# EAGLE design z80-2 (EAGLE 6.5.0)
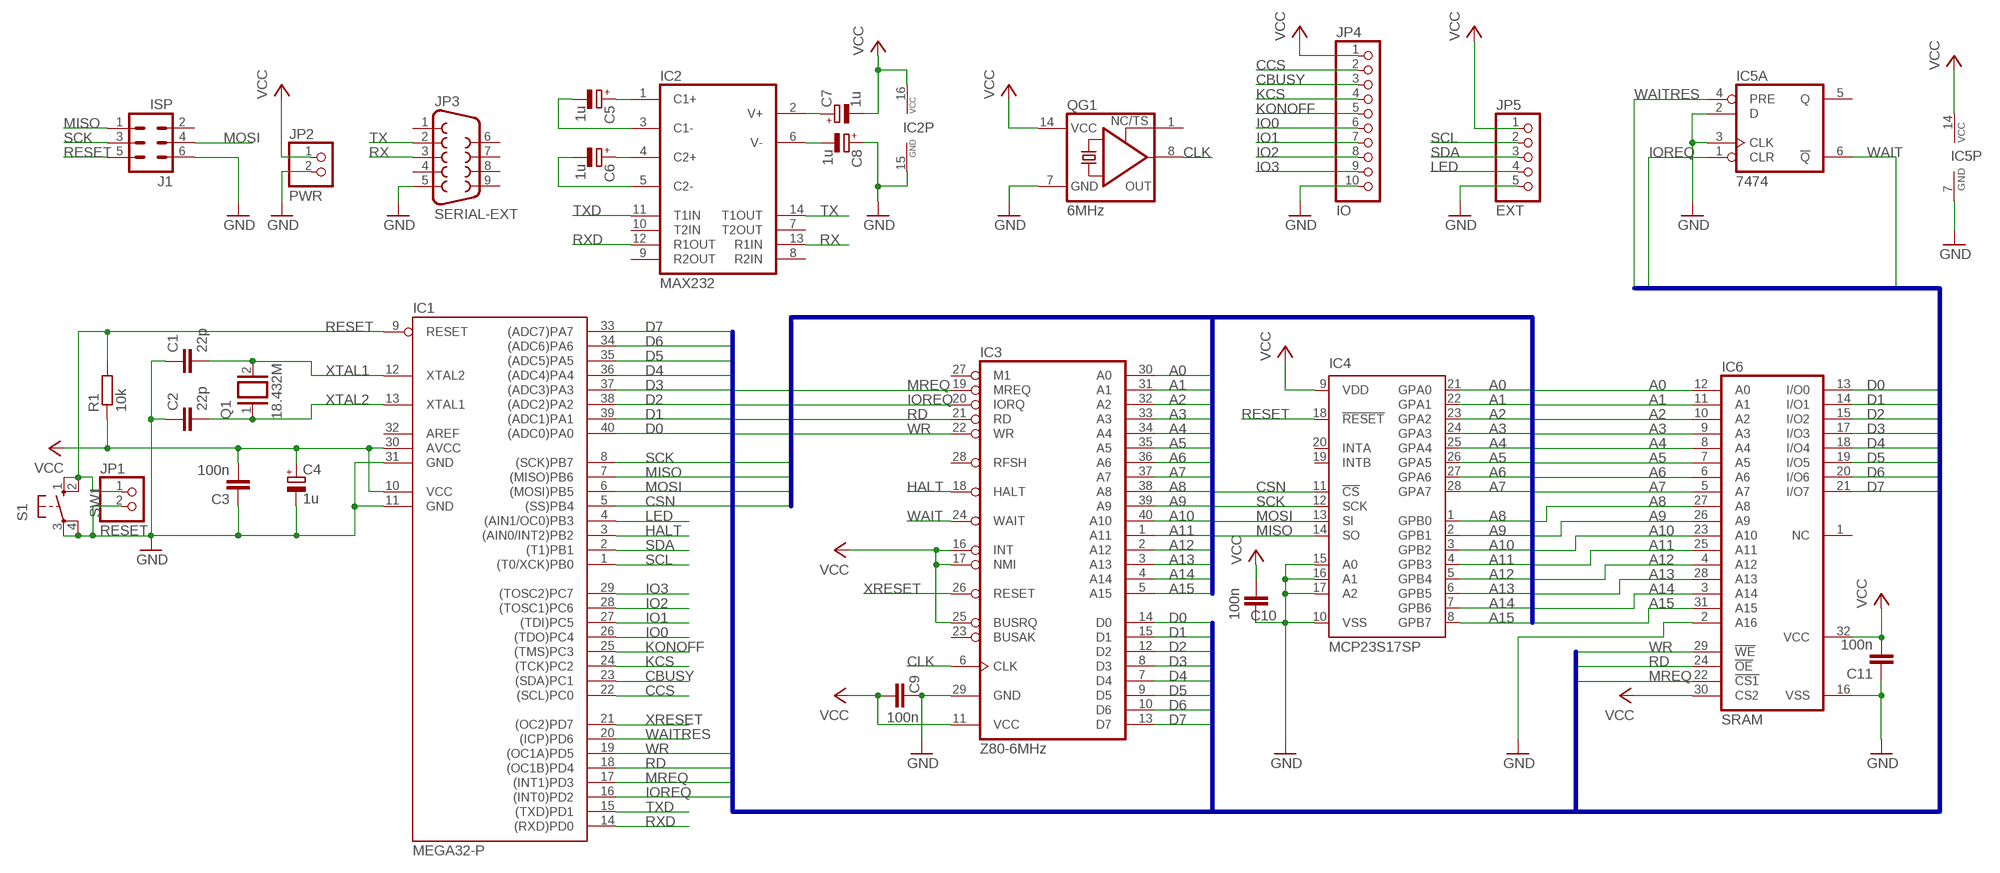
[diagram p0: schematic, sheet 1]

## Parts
C1  22p  C-EU025-024X044  [C025-024X044]
C2  22p  C-EU025-024X044  [C025-024X044]
C3  100n  C-EU025-024X044  [C025-024X044]
C4  1u  CPOL-EUE2.5-5  [E2,5-5]
C5  1u  CPOL-EUE2-5  [E2-5]
C6  1u  CPOL-EUE2.5-5  [E2,5-5]
C7  1u  CPOL-EUE2.5-5  [E2,5-5]
C8  1u  CPOL-EUE2.5-5  [E2,5-5]
C9  100n  C-EU025-024X044  [C025-024X044]
C10  100n  C-EU025-024X044  [C025-024X044]
C11  100n  C-EU025-024X044  [C025-024X044]
IC1  MEGA32-P  [DIL40]
IC2  MAX232  [DIL16]
IC3  Z80-6MHz  Z80CPU  [DIL40]
IC4  MCP23S17SP  [DIL28-3]
IC5  7474  74S74N  [DIL14]
IC6  SRAM  628128P  [DIL32]
J1  ISP  ML6L  [ML6L]
JP1  RESET  PINHD-1X2  [1X02]
JP2  PWR  PINHD-1X2  [1X02]
JP3  SERIAL-EXT  F09HP  [F09HP]
JP4  IO  PINHD-1X10  [1X10]
JP5  EXT  PINHD-1X5  [1X05]
Q1  18.432M  XTAL/S  [QS]
QG1  6MHz  XO-14  [DIL14S]
R1  10k  R-EU_0207/10  [0207/10]
S1  SW1  10-XX  [B3F-10XX]

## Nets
A0: IC3.30(A0) IC4.21(GPA0) IC6.12(A0)
A1: IC3.31(A1) IC4.22(GPA1) IC6.11(A1)
A2: IC3.32(A2) IC4.23(GPA2) IC6.10(A2)
A3: IC3.33(A3) IC4.24(GPA3) IC6.9(A3)
A4: IC3.34(A4) IC4.25(GPA4) IC6.8(A4)
A5: IC3.35(A5) IC4.26(GPA5) IC6.7(A5)
A6: IC3.36(A6) IC4.27(GPA6) IC6.6(A6)
A7: IC3.37(A7) IC4.28(GPA7) IC6.5(A7)
A8: IC3.38(A8) IC4.1(GPB0) IC6.27(A8)
A9: IC3.39(A9) IC4.2(GPB1) IC6.26(A9)
A10: IC3.40(A10) IC4.3(GPB2) IC6.23(A10)
A11: IC3.1(A11) IC4.4(GPB3) IC6.25(A11)
A12: IC3.2(A12) IC4.5(GPB4) IC6.4(A12)
A13: IC3.3(A13) IC4.6(GPB5) IC6.28(A13)
A14: IC3.4(A14) IC4.7(GPB6) IC6.3(A14)
A15: IC3.5(A15) IC4.8(GPB7) IC6.31(A15)
CBUSY: IC1.23((SDA)PC1) JP4.3
CCS: IC1.22((SCL)PC0) JP4.2
CLK: IC3.6(CLK) QG1.8(OUT)
CSN: IC1.5((SS)PB4) IC4.11(!CS)
D0: IC1.40((ADC0)PA0) IC3.14(D0) IC6.13(I/O0)
D1: IC1.39((ADC1)PA1) IC3.15(D1) IC6.14(I/O1)
D2: IC1.38((ADC2)PA2) IC3.12(D2) IC6.15(I/O2)
D3: IC1.37((ADC3)PA3) IC3.8(D3) IC6.17(I/O3)
D4: IC1.36((ADC4)PA4) IC3.7(D4) IC6.18(I/O4)
D5: IC1.35((ADC5)PA5) IC3.9(D5) IC6.19(I/O5)
D6: IC1.34((ADC6)PA6) IC3.10(D6) IC6.20(I/O6)
D7: IC1.33((ADC7)PA7) IC3.13(D7) IC6.21(I/O7)
GND: C1.1 C2.1 C3.1 C4.- C8.+ C9.1 C10.1 C11.1 IC1.11(GND) IC1.31(GND) IC2.15(GND) IC3.29(GND) IC4.10(VSS) IC4.15(A0) IC4.16(A1) IC4.17(A2) IC5.2(A:D) IC5.3(A:CLK) IC5.7(P:GND) IC6.2(A16) IC6.16(VSS) J1.6 JP1.2 JP2.2 JP3.5 JP4.10 JP5.5 QG1.7(GND) S1.3(P) S1.4(P1)
HALT: IC1.3((AIN0/INT2)PB2) IC3.18(HALT)
IO0: IC1.26((TDO)PC4) JP4.6
IO1: IC1.27((TDI)PC5) JP4.7
IO2: IC1.28((TOSC1)PC6) JP4.8
IO3: IC1.29((TOSC2)PC7) JP4.9
IOREQ: IC1.16((INT0)PD2) IC3.20(IORQ) IC5.1(A:CLR)
KCS: IC1.24((TCK)PC2) JP4.4
KONOFF: IC1.25((TMS)PC3) JP4.5
LED: IC1.4((AIN1/OC0)PB3) JP5.4
MISO: IC1.7((MISO)PB6) IC4.14(SO) J1.1
MOSI: IC1.6((MOSI)PB5) IC4.13(SI) J1.4
MREQ: IC1.17((INT1)PD3) IC3.19(MREQ) IC6.22(!CS1)
N$21: C5.+ IC2.1(C1+)
N$22: C6.+ IC2.4(C2+)
N$23: C5.- IC2.3(C1-)
N$24: C6.- IC2.5(C2-)
N$28: C7.+ IC2.2(V+)
N$29: C8.- IC2.6(V-)
RD: IC1.18((OC1B)PD4) IC3.21(RD) IC6.24(!OE)
RESET: IC1.9(RESET) IC4.18(!RESET) J1.5 JP1.1 R1.2 S1.1(S) S1.2(S1)
RX: IC2.13(R1IN) JP3.3
RXD: IC1.14((RXD)PD0) IC2.12(R1OUT)
SCK: IC1.8((SCK)PB7) IC4.12(SCK) J1.3
SCL: IC1.1((T0/XCK)PB0) JP5.2
SDA: IC1.2((T1)PB1) JP5.3
TX: IC2.14(T1OUT) JP3.2
TXD: IC1.15((TXD)PD1) IC2.11(T1IN)
VCC: C3.2 C4.+ C7.- C9.2 C10.2 C11.2 IC1.10(VCC) IC1.30(AVCC) IC2.16(VCC) IC3.11(VCC) IC3.16(INT) IC3.17(NMI) IC3.25(BUSRQ) IC4.9(VDD) IC5.14(P:VCC) IC6.30(CS2) IC6.32(VCC) JP2.1 JP4.1 JP5.1 QG1.14(VCC) R1.1
WAIT: IC3.24(WAIT) IC5.6(A:!Q)
WAITRES: IC1.20((ICP)PD6) IC5.4(A:PRE)
WR: IC1.19((OC1A)PD5) IC3.22(WR) IC6.29(!WE)
XRESET: IC1.21((OC2)PD7) IC3.26(RESET)
XTAL1: C1.2 IC1.12(XTAL2) Q1.2
XTAL2: C2.2 IC1.13(XTAL1) Q1.1
Unconnected: IC1.32(AREF) IC2.7(T2OUT) IC2.8(R2IN) IC2.9(R2OUT) IC2.10(T2IN) IC3.23(BUSAK) IC3.27(M1) IC3.28(RFSH) IC4.19(INTB) IC4.20(INTA) IC5.5(A:Q) IC5.8(B:!Q) IC5.9(B:Q) IC5.10(B:PRE) IC5.11(B:CLK) IC5.12(B:D) IC5.13(B:CLR) IC6.1(NC) J1.2 JP3.1 JP3.4 JP3.6 JP3.7 JP3.8 JP3.9 QG1.1(TS)

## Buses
BUS_ADDR:A[0..15],SCK,MISO,MOSI,CSN
BUD_DAT:D[0..7],RD,WR,MREQ,IOREQ,WAITRES,WAIT

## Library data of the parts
C1-C3 C9-C11 = rcl:C-EU: CAPACITOR, European symbol
C4-C8 = rcl:CPOL-EU: POLARIZED CAPACITOR, European symbol
IC1 = atmel:MEGA32-P: MICROCONTROLLER 32 Kbytes FLASH 2 Kbytes SRAM 1 Kbytes EEPROM USART 8-channel 10 bit ADC Source: www.atmel.com .. doc2503.pdf; MPN: ATMEGA32-16PU; OC_FARNELL: 1661729; OC_NEWARK: 51P1794
IC2 = maxim:MAX232: RS232 TRANSCEIVER; MF: MAXIM; MPN: MAX232ACPE+; OC_FARNELL: 9723773; OC_NEWARK: 68K4544
IC3 = zilog:Z80CPU: Z80 FAMILY DEVICE
IC4 = microchip:MCP23S17: http://ww1.microchip.com/downloads/en/DeviceDoc/21952a.pdf Source: http://ww1.microchip.com/downloads/en/DeviceDoc/21952a.pdf; MF: MICROCHIP; MPN: MCP23S17-E/SP; OC_FARNELL: 1292238; OC_NEWARK: 31K2951
IC5 = 74xx-eu:74*74: Dual D type positive edge triggered FLIP FLOP, preset and clear
IC6 = memory-hitachi:628128P: MEMORY
J1 = con-harting-ml:ML6: HARTING; OC_FARNELL: unknown; OC_NEWARK: unknown
JP1 JP2 = pinhead:PINHD-1X2: PIN HEADER
JP3 = con-subd:F09: SUB-D; OC_FARNELL: unknown; OC_NEWARK: unknown
JP4 = pinhead:PINHD-1X10: PIN HEADER
JP5 = pinhead:PINHD-1X5: PIN HEADER
Q1 = special:XTAL/S: CRYSTAL
QG1 = crystal:XO-: CRYSTAL; OC_FARNELL: unknown; OC_NEWARK: unknown
R1 = rcl:R-EU_: RESISTOR, European symbol
S1 = switch-omron:10-XX: OMRON SWITCH; MPN: B3F-1000; OC_FARNELL: 176432; OC_NEWARK: 36M3542

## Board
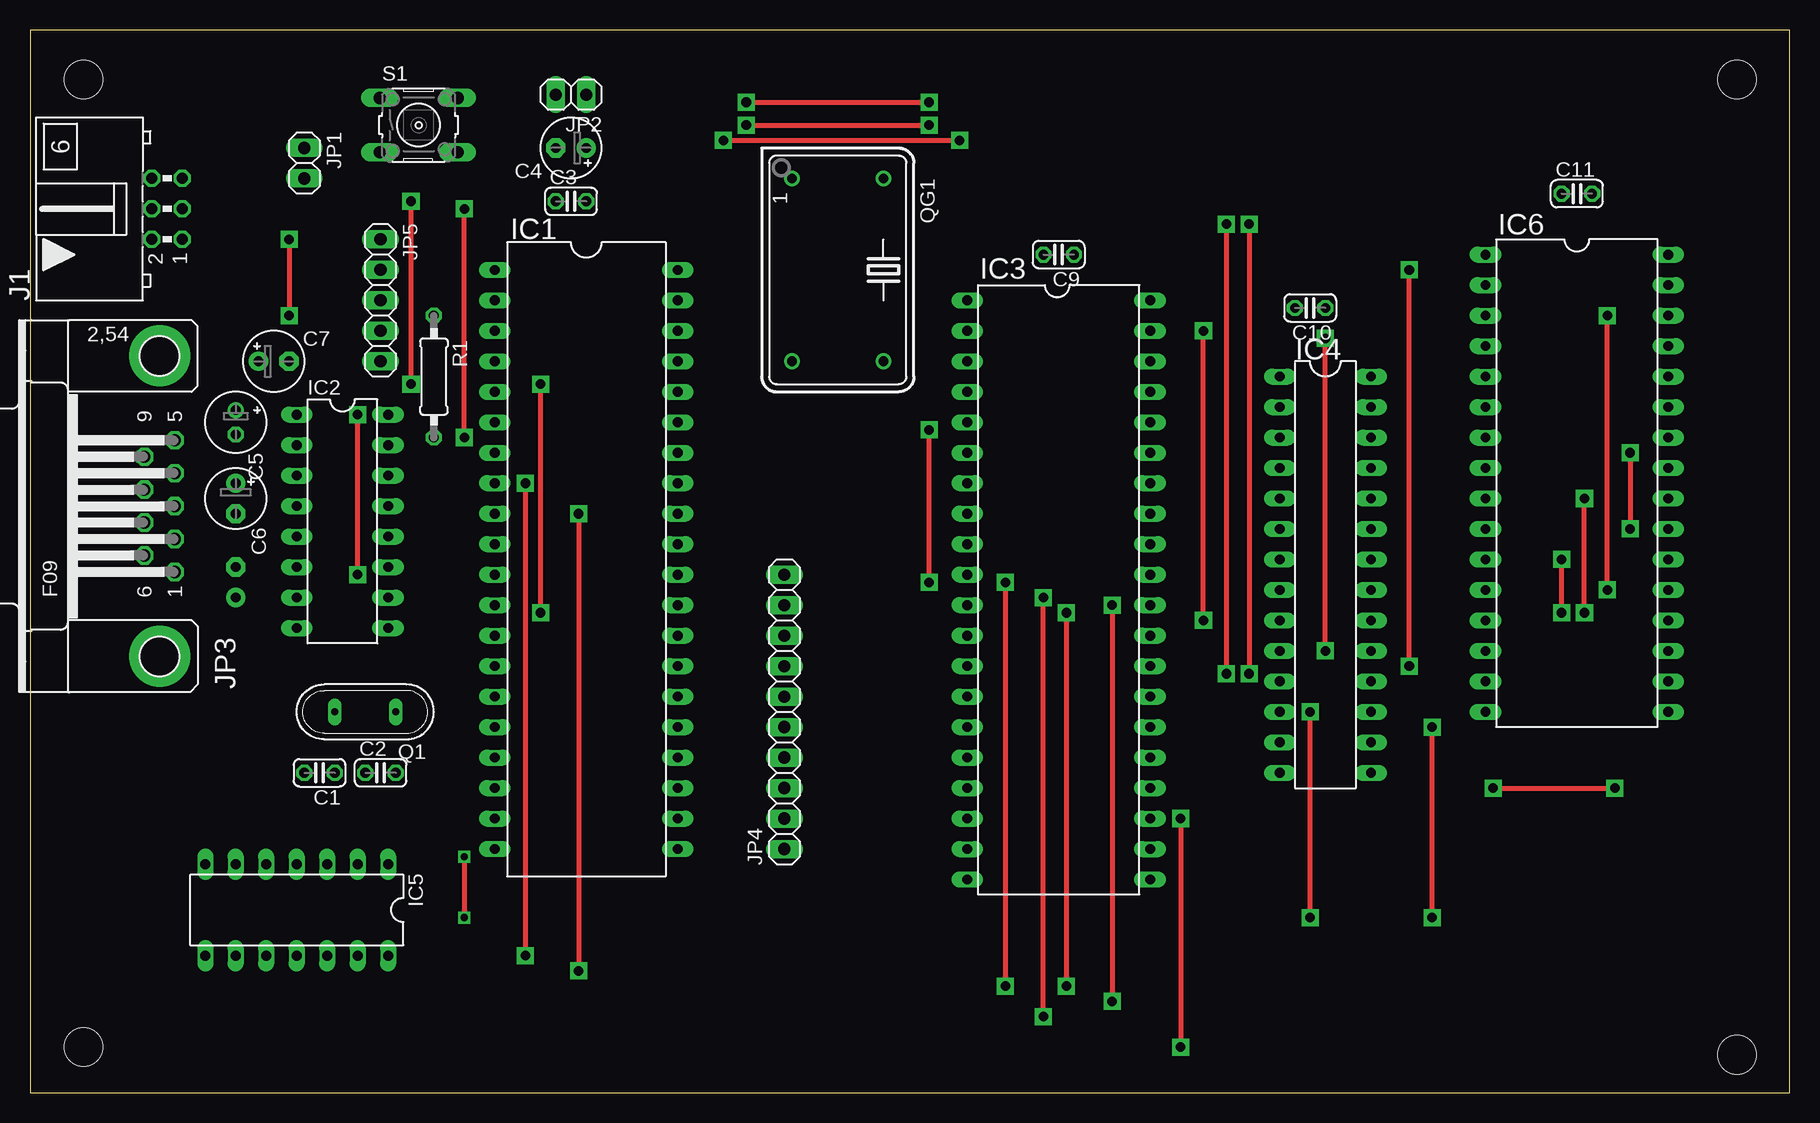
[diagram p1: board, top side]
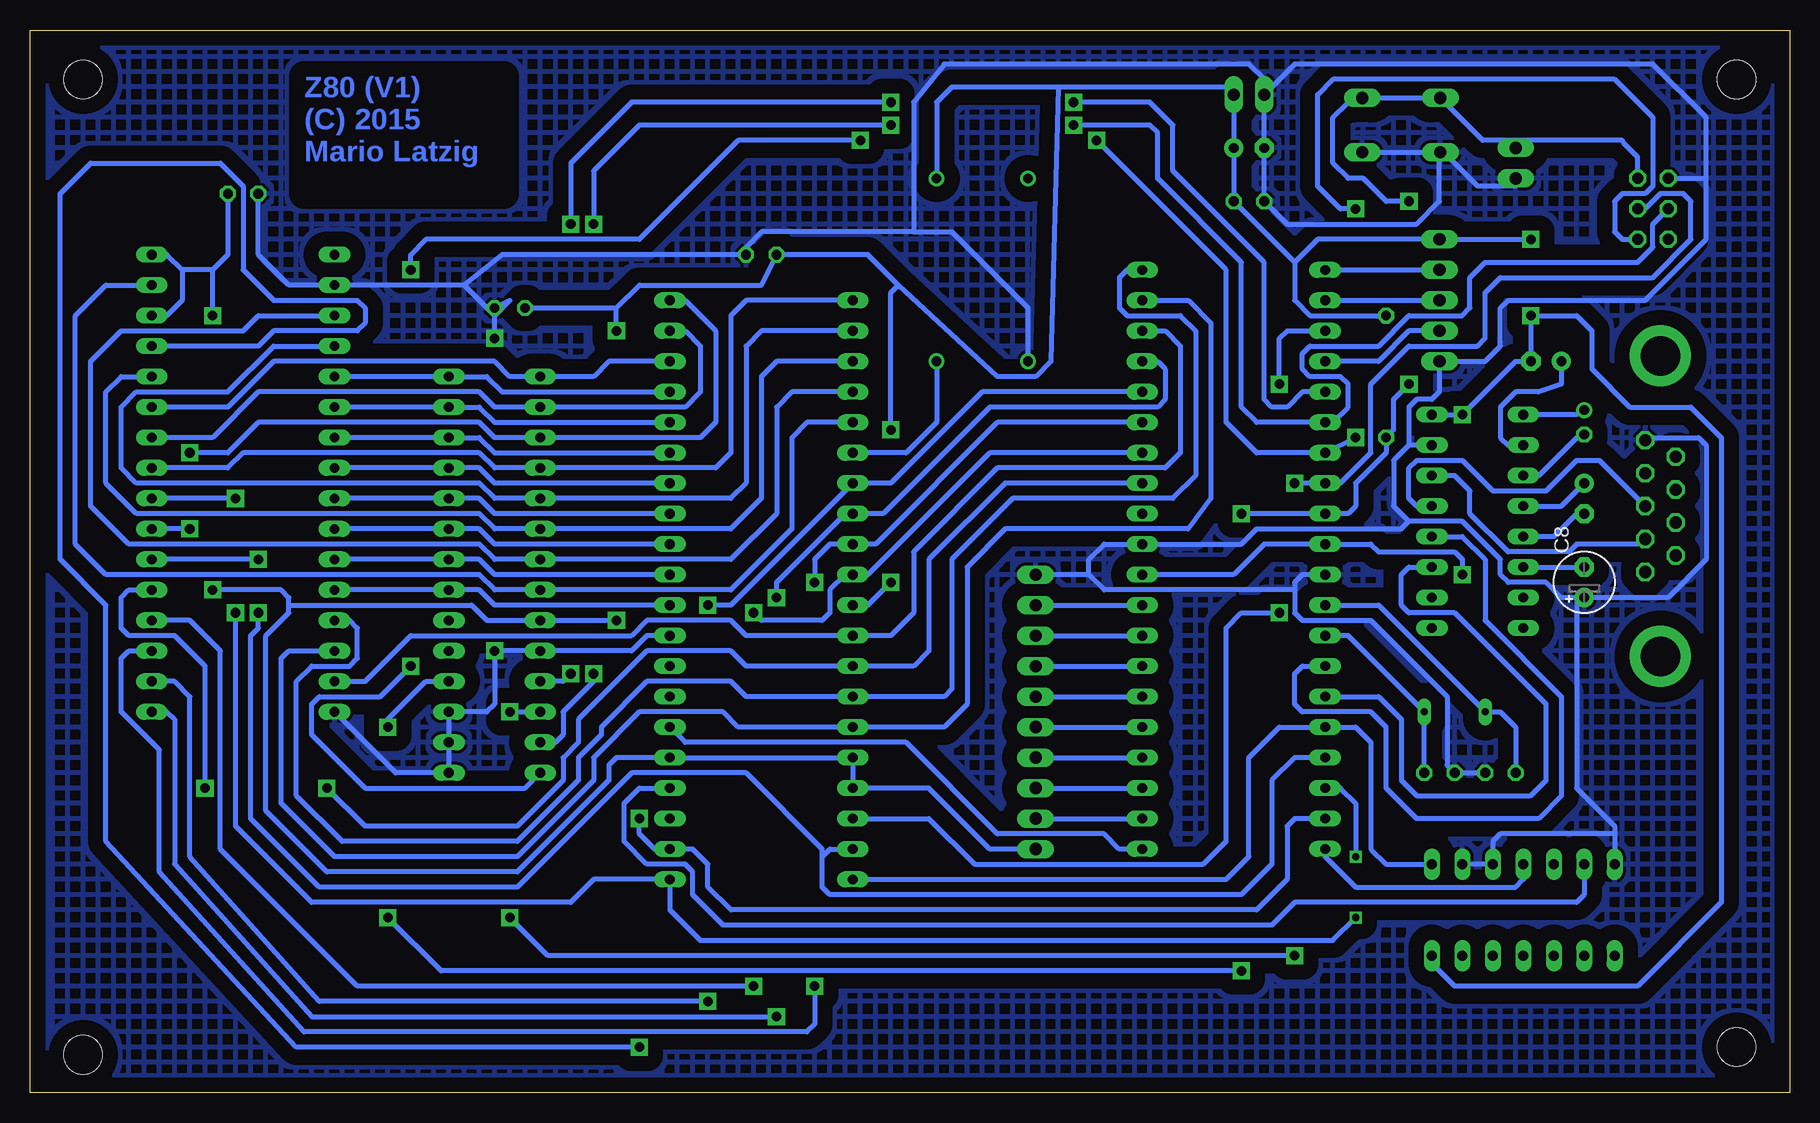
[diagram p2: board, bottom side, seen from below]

Size 146.66 x 88.57 mm. Coordinates in mm from the lower left corner, seen from the top.
Outline: 0,0 146.66,0 146.66,88.57 0,88.57 0,0
Copper layers (1*16): Top 0.035mm / dielectric 1.5mm / Bottom 0.035mm
Design rules "platinenbelichter": minimum track width 10mil, minimum drill 24mil, track to track 10mil, track to pad 10mil, pad to pad 10mil, via to via 10mil, smd to smd 10mil, copper to edge 40mil, drill to drill 8mil, minimum pad ring 10mil, minimum via ring 8mil, stop-mask expansion 10mil, vias tented up to drill 0mil, thermal gap 10mil
Holes 3.2 mm at 4.45,84.45 4.45,3.81 142.24,3.17 142.24,84.45

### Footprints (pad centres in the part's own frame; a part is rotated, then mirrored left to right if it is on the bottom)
C025-024X044 = drill 0.813 octagon: 1 -1.27,0; 2 1.27,0
E2,5-5 = drill 0.813 pad 1.6: + -1.27,0 | drill 0.813 pad 1.6 octagon: - 1.27,0
E2-5 = drill 0.813 pad 1.27: + -1.016,0 | drill 0.813 pad 1.27 octagon: - 1.016,0
DIL40 = drill 0.813 long: 1 -24.13,-7.62; 2 -21.59,-7.62; 3 -19.05,-7.62; 4 -16.51,-7.62; 5 -13.97,-7.62; 6 -11.43,-7.62; 7 -8.89,-7.62; 8 -6.35,-7.62; 9 -3.81,-7.62; 10 -1.27,-7.62; 11 1.27,-7.62; 12 3.81,-7.62; 13 6.35,-7.62; 14 8.89,-7.62; 15 11.43,-7.62; 16 13.97,-7.62; 17 16.51,-7.62; 18 19.05,-7.62; 19 21.59,-7.62; 20 24.13,-7.62; 21 24.13,7.62; 22 21.59,7.62; 23 19.05,7.62; 24 16.51,7.62; 25 13.97,7.62; 26 11.43,7.62; 27 8.89,7.62; 28 6.35,7.62; 29 3.81,7.62; 30 1.27,7.62; 31 -1.27,7.62; 32 -3.81,7.62; 33 -6.35,7.62; 34 -8.89,7.62; 35 -11.43,7.62; 36 -13.97,7.62; 37 -16.51,7.62; 38 -19.05,7.62; 39 -21.59,7.62; 40 -24.13,7.62
DIL16 = drill 0.813 long: 1 -8.89,-3.81; 2 -6.35,-3.81; 3 -3.81,-3.81; 4 -1.27,-3.81; 5 1.27,-3.81; 6 3.81,-3.81; 7 6.35,-3.81; 8 8.89,-3.81; 9 8.89,3.81; 10 6.35,3.81; 11 3.81,3.81; 12 1.27,3.81; 13 -1.27,3.81; 14 -3.81,3.81; 15 -6.35,3.81; 16 -8.89,3.81
DIL28-3 = drill 0.813 long: 1 -16.51,-3.81; 2 -13.97,-3.81; 3 -11.43,-3.81; 4 -8.89,-3.81; 5 -6.35,-3.81; 6 -3.81,-3.81; 7 -1.27,-3.81; 8 1.27,-3.81; 9 3.81,-3.81; 10 6.35,-3.81; 11 8.89,-3.81; 12 11.43,-3.81; 13 13.97,-3.81; 14 16.51,-3.81; 15 16.51,3.81; 16 13.97,3.81; 17 11.43,3.81; 18 8.89,3.81; 19 6.35,3.81; 20 3.81,3.81; 21 1.27,3.81; 22 -1.27,3.81; 23 -3.81,3.81; 24 -6.35,3.81; 25 -8.89,3.81; 26 -11.43,3.81; 27 -13.97,3.81; 28 -16.51,3.81
DIL14 = drill 0.813 long: 1 -7.62,-3.81; 2 -5.08,-3.81; 3 -2.54,-3.81; 4 0,-3.81; 5 2.54,-3.81; 6 5.08,-3.81; 7 7.62,-3.81; 8 7.62,3.81; 9 5.08,3.81; 10 2.54,3.81; 11 0,3.81; 12 -2.54,3.81; 13 -5.08,3.81; 14 -7.62,3.81
DIL32 = drill 0.813 long: 1 -19.05,-7.62; 2 -16.51,-7.62; 3 -13.97,-7.62; 4 -11.43,-7.62; 5 -8.89,-7.62; 6 -6.35,-7.62; 7 -3.81,-7.62; 8 -1.27,-7.62; 9 1.27,-7.62; 10 3.81,-7.62; 11 6.35,-7.62; 12 8.89,-7.62; 13 11.43,-7.62; 14 13.97,-7.62; 15 16.51,-7.62; 16 19.05,-7.62; 17 19.05,7.62; 18 16.51,7.62; 19 13.97,7.62; 20 11.43,7.62; 21 8.89,7.62; 22 6.35,7.62; 23 3.81,7.62; 24 1.27,7.62; 25 -1.27,7.62; 26 -3.81,7.62; 27 -6.35,7.62; 28 -8.89,7.62; 29 -11.43,7.62; 30 -13.97,7.62; 31 -16.51,7.62; 32 -19.05,7.62
ML6L = drill 0.914 octagon: 1 -2.54,-1.27; 2 -2.54,1.27; 3 0,-1.27; 4 0,1.27; 5 2.54,-1.27; 6 2.54,1.27
1X02 = drill 1.016 long: 1 -1.27,0; 2 1.27,0
F09HP = drill 1.016 octagon: 1 -5.486,-1.27; 2 -2.743,-1.27; 3 0,-1.27; 4 2.743,-1.27; 5 5.486,-1.27; 6 -4.115,1.27; 7 -1.372,1.27; 8 1.372,1.27; 9 4.115,1.27 | drill 3.302 pad 5.08: G1 -12.522,0; G2 12.522,0
1X10 = drill 1.016 long: 1 -11.43,0; 2 -8.89,0; 3 -6.35,0; 4 -3.81,0; 5 -1.27,0; 6 1.27,0; 7 3.81,0; 8 6.35,0; 9 8.89,0; 10 11.43,0
1X05 = drill 1.016 long: 1 -5.08,0; 2 -2.54,0; 3 0,0; 4 2.54,0; 5 5.08,0
QS = drill 0.61 long: 1 -2.54,0; 2 2.54,0
DIL14S = drill 0.813: 1 -7.62,-3.81; 7 7.62,-3.81; 8 7.62,3.81; 14 -7.62,3.81
0207/10 = drill 0.813 octagon: 1 -5.08,0; 2 5.08,0
B3F-10XX = drill 1.016 long: 1 -3.251,2.261; 2 3.251,2.261; 3 -3.251,-2.261; 4 3.251,-2.261

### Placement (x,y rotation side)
C1  24.13,26.67 180 top
C2  29.21,26.67 0 top
C3  45.09,74.3 0 top
C4  45.09,78.74 180 top
C5  17.14,55.88 270 top
C6  17.14,49.53 270 top
C7  20.32,60.96 0 top
C8  17.14,42.55 90 bottom
C9  85.72,69.85 180 top
C10  106.68,65.41 180 top
C11  128.91,74.93 0 top
IC1  46.35,44.45 270 top
IC2  26.04,47.62 270 top
IC3  85.72,41.91 270 top
IC4  107.95,43.18 270 top
IC5  22.23,15.24 180 top
IC6  128.91,50.8 270 top
J1  11.43,73.66 90 top
JP1  22.86,77.47 270 top
JP2  45.09,83.19 180 top
JP3  10.79,48.9 90 top
JP4  62.87,31.75 90 top
JP5  29.21,66.04 270 top
Q1  27.94,31.75 180 top
QG1  67.31,68.58 270 top
R1  33.66,59.69 270 top
S1  32.38,80.64 0 top

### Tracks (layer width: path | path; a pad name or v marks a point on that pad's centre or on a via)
A0
  Bottom 0.406: IC6.12 IC4.21 109.22,41.91 107.95,40.64 IC3.30
A1
  Bottom 0.406: IC6.11 IC4.22 109.22,44.45 107.95,43.18 IC3.31
A2
  Bottom 0.406: IC6.10 IC4.23 109.22,46.99 107.95,45.72 IC3.32
A3
  Bottom 0.406: IC6.9 IC4.24 109.22,49.53 107.95,48.26 IC3.33
A4
  Bottom 0.406: IC6.8 IC4.25 109.22,52.07 107.95,50.8 IC3.34
A5
  Bottom 0.406: IC6.7 IC4.26 109.22,54.61 107.95,53.34 IC3.35
A6
  Bottom 0.406: IC6.6 IC4.27 109.22,57.15 107.95,55.88 IC3.36
A7
  Bottom 0.406: IC6.5 IC4.28 108.58,59.69 107.31,58.42 IC3.37
A8
  Bottom 0.406: IC3.38 98.42,60.96 99.69,59.69 IC4.1 106.68,59.69 107.95,60.96 126.36,60.96 130.18,57.15 IC6.27
A9
  Bottom 0.406: IC3.39 92.08,63.5 90.81,62.23 90.81,58.42 92.08,57.15 IC4.2 107.95,57.15 109.22,58.42 127.64,58.42 131.44,54.61 IC6.26
A10  (via drill 0.8 pad 1.42)
  Top 0.406: v133.35,53.34 v133.35,46.99
  Bottom 0.406: IC3.40 92.08,66.04 89.53,63.5 89.53,55.88 90.81,54.61 IC4.3 107.95,54.61 109.22,55.88 127.64,55.88 130.18,53.34 v133.35,53.34 | v133.35,46.99 IC6.23
A11
  Bottom 0.406: IC3.1 87,66.04 88.27,64.77 88.27,53.34 89.53,52.07 IC4.4 107.95,52.07 109.22,53.34 128.91,53.34 130.18,52.07 IC6.25
A12
  Bottom 0.406: IC3.2 85.72,63.5 87,62.23 87,50.8 88.27,49.53 IC4.5 107.95,49.53 109.22,50.8 137.79,50.8 139.06,52.07 139.06,57.15 137.79,58.42 130.18,58.42 126.36,62.23 IC6.4
A13
  Bottom 0.406: IC3.3 84.45,60.96 85.72,59.69 85.72,49.53 88.27,46.99 IC4.6 107.95,46.99 109.22,48.26 137.79,48.26 140.34,50.8 140.34,58.42 139.06,59.69 IC6.28
A14
  Bottom 0.406: IC3.4 83.19,58.42 84.45,57.15 84.45,48.26 88.27,44.45 IC4.7 107.95,44.45 109.22,45.72 138.43,45.72 141.6,48.9 141.6,60.96 139.06,63.5 128.91,63.5 127.64,64.77 IC6.3
A15
  Bottom 0.406: IC3.5 81.92,55.88 83.19,54.61 83.19,46.99 88.27,41.91 IC4.8 107.95,41.91 109.22,43.18 140.34,43.18 142.88,45.72 142.88,64.77 140.34,67.31 IC6.31
CBUSY
  Bottom 0.406: JP4.3 IC1.23
CCS
  Bottom 0.406: JP4.2 IC1.22
CLK
  Bottom 0.406: QG1.8 71.12,55.88 73.66,53.34 IC3.6
CSN  (via drill 0.8 pad 1.42)
  Top 0.406: v59.69,82.55 v74.93,82.55 | v101.6,72.39 v101.6,34.92
  Bottom 0.406: IC1.5 40.64,58.42 41.91,57.15 43.18,57.15 43.81,57.78 43.81,69.22 51.44,76.83 51.44,80.64 53.34,82.55 v59.69,82.55 | v74.93,82.55 96.52,82.55 101.6,77.47 v101.6,72.39 | v101.6,34.92 102.23,34.29 IC4.11
D0
  Bottom 0.406: IC6.13 120.02,39.37 119.38,38.73 119.38,36.2 120.02,35.56 123.19,35.56 124.46,34.29 124.46,24.77 120.65,20.95 106.05,20.95 100.97,26.04 100.97,27.94 99.06,29.84 99.06,30.48 95.25,34.29 88.27,34.29 87,33.02 IC3.14 70.48,33.02 69.85,33.66 69.85,44.45 64.77,49.53 51.44,49.53 49.53,51.44 49.53,63.5 50.8,64.77 55.24,64.77 55.88,65.41 55.88,67.94 55.24,68.58 IC1.40
D1
  Bottom 0.406: IC6.14 125.09,36.83 125.73,36.2 125.73,24.13 121.28,19.68 106.05,19.68 99.69,26.04 99.69,27.94 95.89,31.75 88.9,31.75 87.63,30.48 IC3.15 70.48,30.48 68.58,32.38 68.58,43.81 65.41,46.99 50.16,46.99 48.26,49.53 48.26,64.14 50.16,66.04 IC1.39
D2
  Bottom 0.406: IC1.38 52.07,63.5 50.8,62.23 50.8,53.34 52.07,52.07 66.04,52.07 73.03,45.09 73.03,40.01 74.93,38.1 IC3.12 87,38.1 88.27,39.37 95.25,39.37 96.52,38.1 114.94,38.1 118.75,34.29 IC6.15
D3  (via drill 0.8 pad 1.42)
  Top 0.406: v84.45,6.35 v84.45,41.27
  Bottom 0.406: IC6.17 135.25,31.75 134.62,31.11 134.62,19.05 123.19,6.35 v84.45,6.35 | v84.45,41.27 84.45,42.55 78.74,48.26 IC3.8 75.56,48.26 66.67,57.15 52.7,57.15 52.07,57.78 52.07,60.33 52.7,60.96 IC1.37
D4  (via drill 0.8 pad 1.42)
  Top 0.406: v90.17,40.64 v90.17,7.62
  Bottom 0.406: v90.17,40.64 88.27,40.64 IC3.7 74.93,50.8 67.31,58.42 IC1.36 | v90.17,7.62 122.56,7.62 133.35,19.68 133.35,33.02 134.62,34.29 IC6.18
D5  (via drill 0.8 pad 1.42)
  Top 0.406: v81.28,42.55 v81.28,8.89
  Bottom 0.406: v81.28,42.55 81.28,44.45 80.01,45.72 IC3.9 76.2,45.72 66.04,55.88 IC1.35 | v81.28,8.89 81.28,5.71 81.92,5.08 123.83,5.08 135.89,18.41 135.89,28.57 139.06,31.75 139.06,36.2 138.43,36.83 IC6.19
D6  (via drill 0.8 pad 1.42)
  Top 0.406: v86.36,40.01 v86.36,8.89
  Bottom 0.406: v86.36,40.01 85.72,39.37 80.64,39.37 80.01,40.01 80.01,41.91 78.74,43.18 IC3.10 76.83,43.18 66.67,53.34 IC1.34 | v86.36,8.89 119.38,8.89 130.81,20.32 130.81,36.83 133.35,39.37 IC6.20
D7  (via drill 0.8 pad 1.42)
  Top 0.406: v121.92,25.4 v132.08,25.4
  Bottom 0.406: v121.92,25.4 118.75,22.23 106.05,22.23 102.23,26.04 102.23,27.94 100.97,29.21 100.97,31.11 95.25,36.83 88.27,36.83 87,35.56 IC3.13 73.03,35.56 71.75,36.83 71.75,44.45 65.41,50.8 IC1.33 | v132.08,25.4 132.08,35.56 134.62,38.1 138.43,38.1 139.06,38.73 139.06,41.27 138.43,41.91 IC6.21
GND  (via drill 0.8 pad 1.42)
  Top 0.406: v107.95,36.83 v107.95,62.87
  Bottom 0.406: C11.1 127.64,69.85 125.09,67.31 IC6.2 110.49,67.31 | IC6.16 116.2,26.67 IC4.15 IC4.16 IC4.17 108.58,31.75 107.95,32.38 v107.95,36.83 IC4.10 96.52,36.83 95.25,38.1 IC3.29 | C1.1 C2.1 28.57,27.3 28.57,33.02 34.92,39.37 40.64,39.37 41.27,40.01 41.27,41.91 | IC1.11 40.64,43.18 41.27,42.55 41.27,41.91 | 17.78,41.27 C8.+ 10.16,41.27 6.99,44.45 6.99,53.98 7.62,54.61 11.43,54.61 JP3.5 | 17.78,41.27 19.05,41.27 20.32,42.55 23.5,42.55 24.13,43.18 24.13,44.45 27.3,47.62 31.75,47.62 | 31.75,47.62 32.38,46.99 44.45,46.99 45.72,45.72 IC1.31 57.15,45.72 58.42,44.45 58.42,43.18 | IC2.15 31.75,53.98 | 31.75,53.98 33.02,52.7 33.02,48.9 31.75,47.62 | 31.75,53.98 31.75,57.15 31.11,57.78 29.84,57.78 29.21,58.42 JP5.5 25.4,60.96 24.13,62.23 24.13,65.41 23.5,66.04 12.06,66.04 6.99,71.12 6.99,76.2 | S1.3 28.85,78.11 28.57,78.11 26.04,75.56 22.86,75.56 JP1.2 | JP2.2 C4.- C3.1 41.91,72.39 31.11,72.39 29.21,74.3 29.21,78.31 S1.3 | JP2.2 43.81,84.45 45.09,85.72 70.48,85.72 73.03,82.55 73.03,71.75 | 73.03,71.75 69.85,71.75 63.5,65.41 QG1.7 | S1.4 S1.3 | 6.99,76.2 6.99,81.28 11.43,85.72 41.27,85.72 JP2.2 | 41.27,41.91 57.15,41.91 58.42,43.18 | 58.42,43.18 JP4.10 | 73.03,71.75 85.72,71.75 87,70.48 C9.1 107.31,69.85 110.49,67.31 | v107.95,62.87 107.95,64.77 | 107.95,64.77 110.49,67.31 | C10.1 106.68,66.04 107.95,64.77 | J1.6 6.99,76.2 | 17.78,41.27 17.78,25.4 14.61,22.23 14.61,21.59 | 14.61,21.59 IC5.7 | 14.61,21.59 24.13,21.59 24.77,20.95 IC5.3 IC5.2
  pour Bottom (isolate 1.27, hatched): 146.69,88.9 146.69,0 0,0 0,88.9
HALT  (via drill 0.8 pad 1.42)
  Top 0.406: v42.55,40.01 v42.55,59.05
  Bottom 0.406: IC3.18 71.75,22.86 67.94,19.05 48.9,19.05 46.99,20.95 46.99,38.73 45.72,40.01 v42.55,40.01 | v42.55,59.05 42.55,62.87 41.91,63.5 IC1.3
IO0
  Bottom 0.406: JP4.6 IC1.26
IO1
  Bottom 0.406: JP4.7 IC1.27
IO2
  Bottom 0.406: JP4.8 IC1.28
IO3
  Bottom 0.406: JP4.9 IC1.29
IOREQ
  Bottom 0.406: IC3.20 46.99,17.78 45.09,19.68 45.09,27.94 42.55,30.48 IC1.16 36.2,30.48 34.92,29.21 34.92,20.32 33.66,19.05 IC5.1
KCS
  Bottom 0.406: JP4.4 IC1.24
KONOFF
  Bottom 0.406: JP4.5 IC1.25
LED
  Bottom 0.406: JP5.4 31.75,63.5 34.29,60.96 IC1.4
MISO  (via drill 0.8 pad 1.42)
  Top 0.406: v36.2,54.61 v36.2,73.66 | v57.78,79.38 v77.47,79.38 | v114.94,35.56 v114.94,68.58
  Bottom 0.406: v36.2,54.61 IC1.7 44.45,53.34 46.99,55.88 46.99,68.58 v57.78,79.38 | v36.2,73.66 37.47,73.66 39.37,75.56 39.37,83.19 38.1,84.45 14.61,84.45 11.43,81.28 11.43,75.56 12.06,74.93 13.97,74.93 14.61,74.3 14.61,71.75 13.97,71.12 J1.1 | v77.47,79.38 87.63,79.38 95.89,71.12 113.67,71.12 114.94,69.85 v114.94,68.58 | IC4.14 105.41,25.4 118.75,25.4 123.19,29.84 123.19,32.38 122.56,33.02 117.47,33.02 v114.94,35.56
MOSI  (via drill 0.8 pad 1.42)
  Top 0.406: v59.69,80.64 v74.93,80.64 | v99.69,72.39 v99.69,34.92
  Bottom 0.406: v59.69,80.64 53.34,80.64 52.7,80.01 52.7,76.2 45.72,69.22 45.72,57.15 44.45,55.88 IC1.6 38.1,55.88 36.83,57.15 36.83,59.05 37.47,59.69 40.01,59.69 40.64,60.33 40.64,61.59 40.01,62.23 34.29,62.23 31.75,64.77 27.3,64.77 26.67,65.41 26.67,67.94 25.4,69.22 12.7,69.22 11.43,70.48 11.43,72.39 J1.4 | v74.93,80.64 95.89,80.64 99.69,76.83 v99.69,72.39 | v99.69,34.92 99.69,34.29 102.23,31.75 102.23,29.84 102.87,29.21 IC4.13
MREQ  (via drill 0.8 pad 1.42)
  Top 0.406: v127.64,40.01 v127.64,44.45
  Bottom 0.406: IC1.17 41.27,27.94 43.18,26.04 43.18,19.05 45.72,16.51 80.01,16.51 80.64,17.14 80.64,19.68 | 80.64,19.68 80.01,20.32 IC3.19 | 80.64,19.68 80.64,20.32 87,26.67 96.52,26.67 106.05,17.14 122.56,17.14 128.27,22.86 128.27,38.1 127.64,38.73 v127.64,40.01 | v127.64,44.45 IC6.22 137.16,44.45
N$21
  Bottom 0.406: C5.+ 17.4,56.9 17.78,56.52 IC2.1
N$22
  Bottom 0.406: IC2.4 19.05,48.9 C6.+
N$23
  Bottom 0.406: IC2.3 20.95,51.44 17.78,54.61 17.4,54.61 C5.-
N$24
  Bottom 0.406: C6.- 17.78,48.26 19.68,46.35 IC2.5
N$28
  Bottom 0.406: C7.+ 19.05,59.05 20.95,58.42 22.86,58.42 24.13,57.15 24.13,54.61 23.5,53.98 IC2.2
N$29
  Bottom 0.406: IC2.6 C8.-
RD  (via drill 0.6, 0.8 pad 1.42)
  Top 0.406: v129.54,40.01 v129.54,49.53 | v36.2,19.68 v36.2,14.61
  Bottom 0.406: v129.54,40.01 129.54,22.23 123.19,15.88 101.6,15.88 99.69,17.78 IC3.21 93.34,15.24 90.81,12.7 38.1,12.7 v36.2,14.61 | v129.54,49.53 IC6.24 | IC1.18 37.47,25.4 36.2,24.13 v36.2,19.68
RESET  (via drill 0.8 pad 1.42)
  Top 0.406: v31.75,59.05 v31.75,74.3 | v45.72,48.26 v45.72,10.16 | v116.84,14.61 v116.84,30.48
  Bottom 0.406: S1.1 S1.2 35.99,82.55 36.83,82.55 38.1,81.28 38.1,77.47 36.83,76.2 35.56,76.2 33.66,74.3 v31.75,74.3 | 28.22,82.55 S1.1 | v31.75,59.05 33.02,57.78 33.02,55.24 R1.2 33.66,53.34 36.2,50.8 36.2,48.9 36.83,48.26 IC1.9 v45.72,48.26 | 22.86,79.38 13.97,79.38 13.84,79.12 12.7,77.98 J1.5 | 22.86,79.38 25.6,79.38 S1.1 | v45.72,10.16 112.39,10.16 v116.84,14.61 | v116.84,30.48 116.84,31.11 113.67,34.29 IC4.18 | JP1.1 22.86,79.38
RX
  Bottom 0.406: IC2.13 31.11,48.9 31.75,49.53 31.75,52.07 31.11,52.7 27.3,52.7 24.77,50.16 20.32,50.16 17.78,52.7 15.88,52.7 JP3.3
RXD
  Bottom 0.406: IC2.12 27.3,46.35 25.4,44.45 25.4,39.37 19.05,33.02 19.05,24.77 20.95,22.86 31.11,22.86 33.66,25.4 33.66,30.48 34.92,31.75 40.64,31.75 41.27,32.38 41.27,34.92 40.64,35.56 IC1.14
SCK  (via drill 0.8 pad 1.42)
  Top 0.406: v41.27,50.8 v41.27,11.43 | v106.68,14.61 v106.68,31.75
  Bottom 0.406: v41.27,50.8 IC1.8 37.47,50.8 34.92,53.34 34.92,59.05 31.75,62.23 26.04,62.23 25.4,62.87 25.4,66.67 24.13,67.94 11.43,67.94 8.26,71.12 8.26,74.3 8.89,74.93 10.79,74.93 12.06,73.66 J1.3 | v41.27,11.43 103.5,11.43 v106.68,14.61 | v106.68,31.75 IC4.12
SCL
  Bottom 0.406: IC1.1 JP5.2
SDA
  Bottom 0.406: IC1.2 JP5.3
TX
  Bottom 0.406: JP3.2 12.27,46.15 12.7,45.72 17.78,45.72 18.41,45.09 23.5,45.09 26.67,48.26 26.67,50.16 27.94,51.44 IC2.14
TXD
  Bottom 0.406: IC1.15 34.29,33.02 32.38,31.11 32.38,26.04 31.11,24.77 21.59,24.77 20.32,26.04 20.32,32.38 27.94,40.01 31.75,40.01 32.38,40.64 32.38,43.18 31.75,43.81 IC2.11
VCC  (via drill 0.8 pad 1.42)
  Top 0.406: v21.59,71.12 v21.59,64.77 | v27.3,43.18 v27.3,56.52 | v74.93,42.55 v74.93,55.24 | v97.79,39.37 v97.79,63.5 | v131.44,41.91 v131.44,64.77
  Bottom 0.406: IC6.32 135.25,69.85 133.99,68.58 | 133.99,68.58 133.99,66.04 135.25,64.77 IC6.30 | C11.2 130.18,69.85 131.44,68.58 | 131.44,68.58 133.99,68.58 | IC1.30 46.35,43.18 43.81,45.72 IC1.10 34.92,45.72 34.29,45.09 27.94,45.09 27.3,44.45 v27.3,43.18 | IC2.16 v27.3,56.52 22.86,60.96 C7.- v21.59,64.77 17.78,64.77 16.51,63.5 16.51,60.33 13.34,57.15 8.26,57.15 5.71,54.61 5.71,15.88 12.7,8.89 27.94,8.89 29.84,10.79 IC5.14 | 41.27,69.22 39.37,71.12 JP5.1 v21.59,71.12 | 41.27,69.22 41.27,66.04 40.01,64.77 R1.1 | JP4.1 66.67,20.32 71.75,25.4 IC3.17 IC3.16 IC3.25 97.79,27.94 98.42,27.3 98.42,26.04 106.05,18.41 121.92,18.41 127,23.5 127,38.1 125.09,40.01 125.09,40.64 | 60.96,83.82 46.99,83.82 JP2.1 C4.+ C3.2 41.27,69.22 | 60.96,83.82 69.85,83.82 71.12,82.55 QG1.14 | 60.96,83.82 61.59,60.96 62.87,59.69 66.04,59.69 74.3,67.31 | 74.3,67.31 76.83,69.85 C9.2 85.72,67.31 95.89,67.31 97.79,65.41 | IC3.11 76.83,40.64 v74.93,42.55 | v74.93,55.24 74.93,66.67 74.3,67.31 | v97.79,39.37 IC4.9 108.58,39.37 109.86,40.64 125.09,40.64 | v97.79,63.5 97.79,65.41 | 125.09,40.64 125.09,41.27 125.73,41.91 v131.44,41.91 | v131.44,64.77 131.44,68.58 | C10.2 97.79,65.41
WAIT
  Bottom 0.406: IC3.24 95.89,25.4 97.16,24.13 97.16,20.95 95.25,19.05 92.08,19.05 91.44,18.41 91.44,16.51 88.9,13.97 43.18,13.97 41.27,15.88 17.78,15.88 17.14,16.51 IC5.6
WAITRES
  Bottom 0.406: IC1.20 38.73,19.68 36.2,17.14 22.86,17.14 22.23,17.78 IC5.4
WR  (via drill 0.8 pad 1.42)
  Top 0.406: v95.89,22.86 v95.89,3.81
  Bottom 0.406: IC1.19 41.27,22.86 41.91,22.23 41.91,17.78 44.45,15.24 88.27,15.24 90.17,17.14 90.17,19.05 91.44,20.32 IC3.22 94.61,20.32 95.89,21.59 v95.89,22.86 | v95.89,3.81 124.46,3.81 140.34,20.95 140.34,40.64 144.15,44.45 144.15,74.93 141.6,77.47 130.81,77.47 128.91,75.56 128.91,68.58 126.36,66.04 119.38,66.04 118.75,65.41 118.75,64.14 119.38,63.5 126.36,63.5 127.64,62.23 IC6.29
XRESET
  Bottom 0.406: IC1.21 55.88,20.32 57.15,21.59 66.04,21.59 73.66,29.21 92.08,29.21 IC3.26
XTAL1
  Bottom 0.406: IC1.12 34.29,40.64 Q1.2 24.13,31.75 22.86,30.48 C1.2
XTAL2
  Bottom 0.406: IC1.13 36.83,38.1 Q1.1 C2.2

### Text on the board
Bottom: Z80 (V1) / (C) 2015 / Mario Latzig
